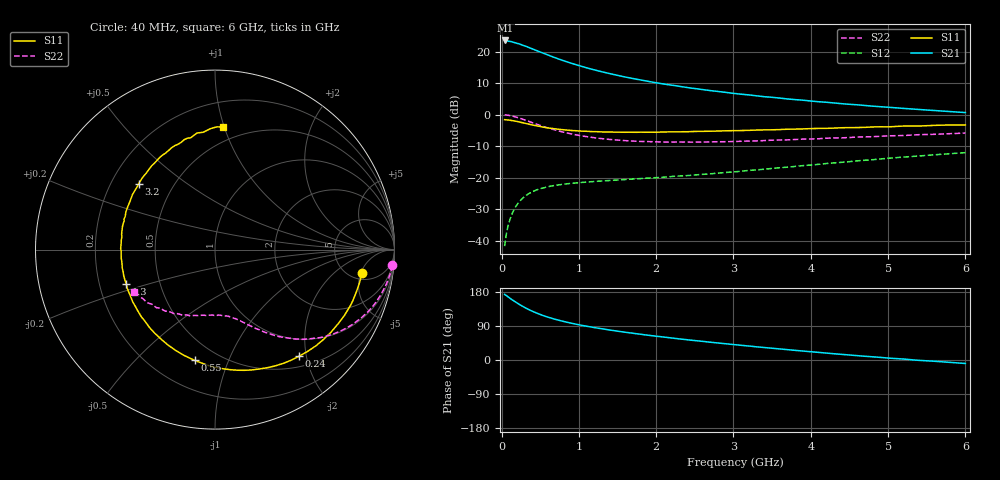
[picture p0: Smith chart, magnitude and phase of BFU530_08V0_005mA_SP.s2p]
! Filename:  P:\Prog\Test\Noise\ATS_data\Testdata_Net\03 Spar\BFU530_APG2013_40_A05_08p0V_005mA_SP_CM01_D.s2p
! Date/Time: Fri 26/Apr/2013 13:03:14
! BFU530_APG2013_40_A05_08p0V_1to25mA_SP_CM01_Bias4_R.s2p
! MDIF S-parameter v. bias file
! BFU530_APG2013_40_A05_08p0V_1to25mA_SP_CM01
! Date/time Wed Apr 24 16:58:28 2013
! VAR V_out= 8.0000
! VAR I_out= 4.9950
! VAR V_in= 0.8132
! VAR I_in= 0.0526
! Device data file deembeded for feedlines and parallel
! Original file: \03 Spar\BFU530_APG2013_40_A05_08p0V_005mA_SP_CM01_R.s2p
! Feed-files: PR047V01_250413_Feed1.s2p, PR047V01_250413_Feed2.s2p
! Parallel-file: PR047V01_250413_Par.s2p
# MHz S MA R 50
!  Freq-MHz  S11-mag  S11-arg  S21-mag  S21-arg  S12-mag  S12-arg  S22-mag  S22-arg
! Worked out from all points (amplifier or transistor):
!   98 points, 40 MHz to 6 GHz, reference 50 ohm
!   highest |S21| = 23.5 dB at 50 MHz (marker M1)
!   |S21| within 3 dB of that: start of sweep to 432.1 MHz
!   unconditionally stable (mu >= 1): 2.269 GHz to 4.35 GHz
!   at 300 MHz: K = 0.19, MSG = 23.9 dB, |S12| = -26.0 dB
!   at 1.6 GHz: K = 0.82, MSG = 16.3 dB, |S12| = -20.6 dB
!   at 6 GHz: K = 0.85, MSG = 6.4 dB, |S12| = -12.1 dB
!   S11 on the Smith chart (normalised r, x): 40 MHz: 6.27, -5.28; 240 MHz: 0.67, -1.87; 550 MHz: 0.37, -0.76; 1.3 GHz: 0.32, -0.17; 3.2 GHz: 0.32, +0.34; 6 GHz: 0.39, +0.99
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40  0.8302 -9.1  14.97 173.4  0.008167 84.9  0.9902 -5.1
50  0.8276 -11.3  14.97 171.4  0.01016 83.6  0.9892 -6.5
140  0.8004 -31.3  14.2 158.6  0.02723 73.3  0.9451 -17.8
220  0.7664 -47.8  13.31 148.0  0.03997 65.2  0.8864 -26.6
240  0.7565 -51.7  13.05 145.5  0.04276 63.3  0.8714 -28.6
320  0.7184 -66.5  12.05 136.4  0.05232 56.8  0.8056 -35.9
360  0.7006 -73.2  11.51 132.4  0.05626 54.1  0.7741 -39.0
460  0.6597 -88.3  10.28 123.4  0.06416 48.4  0.7 -45.6
550  0.6274 -100.5  9.305 116.4  0.06898 44.4  0.6392 -50.4
650  0.6024 -111.6  8.342 110.0  0.07372 41.2  0.5885 -54.8
750  0.5815 -121.5  7.522 104.4  0.077 38.9  0.545 -58.3
900  0.5587 -134.2  6.53 97.2  0.08103 36.4  0.4945 -62.7
1050  0.5448 -144.8  5.747 91.0  0.08394 35.0  0.4563 -66.4
1300  0.5304 -159.1  4.766 82.3  0.08835 33.9  0.4146 -71.5
1600  0.5236 -173.2  3.939 73.2  0.09306 33.9  0.3859 -76.9
2050  0.5271 170.7  3.117 61.7  0.1006 35.3  0.3676 -84.7
2450  0.537 157.9  2.63 52.3  0.1085 36.9  0.3649 -92.0
3100  0.5575 140.9  2.103 38.8  0.1262 39.5  0.377 -102.9
3200  0.5617 139.1  2.049 36.8  0.13 39.8  0.3799 -104.4
4100  0.6025 118.9  1.598 20.1  0.1622 39.8  0.4131 -120.3
5200  0.6574 98.7  1.252 2.5  0.2113 35.4  0.4646 -139.1
6000  0.6848 86.2  1.076 -9.2  0.2487 29.7  0.5084 -152.4
